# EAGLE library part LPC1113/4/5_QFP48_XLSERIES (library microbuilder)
LPC1113/4/5 ARM Cortex M0 MCU (50MHz) - XL Series (FBD48/3x3) LPC1115FBD48/303: Max Frequency: 50MHz Flash: 64kB SRAM: 8kB ADC: 10-bit
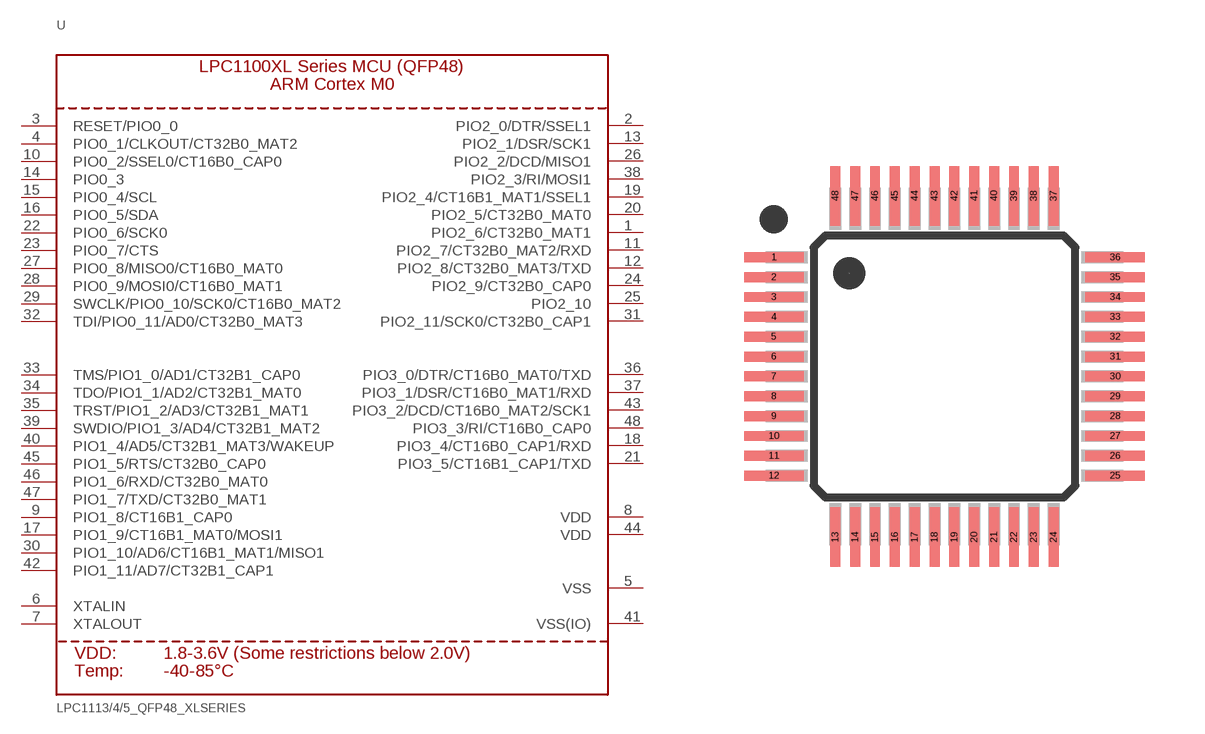
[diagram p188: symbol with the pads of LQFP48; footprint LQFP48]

Designator prefix U

## LPC1113/4/5_QFP48_XLSERIES  [LQFP48]
1  PIO2_6/CT32B0_MAT1
2  PIO2_0/DTR/SSEL1
3  RESET/PIO0_0
4  PIO0_1/CLKOUT/CT32B0_MAT2
5  VSS  pwr
6  XTALIN  in
7  XTALOUT  out
8  VDD  pwr
9  PIO1_8/CT16B1_CAP0
10  PIO0_2/SSEL0/CT16B0_CAP0
11  PIO2_7/CT32B0_MAT2/RXD
12  PIO2_8/CT32B0_MAT3/TXD
13  PIO2_1/DSR/SCK1
14  PIO0_3
15  PIO0_4/SCL
16  PIO0_5/SDA
17  PIO1_9/CT16B1_MAT0/MOSI1
18  PIO3_4/CT16B0_CAP1/RXD
19  PIO2_4/CT16B1_MAT1/SSEL1
20  PIO2_5/CT32B0_MAT0
21  PIO3_5/CT16B1_CAP1/TXD
22  PIO0_6/SCK0
23  PIO0_7/CTS
24  PIO2_9/CT32B0_CAP0
25  PIO2_10
26  PIO2_2/DCD/MISO1
27  PIO0_8/MISO0/CT16B0_MAT0
28  PIO0_9/MOSI0/CT16B0_MAT1
29  SWCLK/PIO0_10/SCK0/CT16B0_MAT2
30  PIO1_10/AD6/CT16B1_MAT1/MISO1
31  PIO2_11/SCK0/CT32B0_CAP1
32  TDI/PIO0_11/AD0/CT32B0_MAT3
33  TMS/PIO1_0/AD1/CT32B1_CAP0
34  TDO/PIO1_1/AD2/CT32B1_MAT0
35  TRST/PIO1_2/AD3/CT32B1_MAT1
36  PIO3_0/DTR/CT16B0_MAT0/TXD
37  PIO3_1/DSR/CT16B0_MAT1/RXD
38  PIO2_3/RI/MOSI1
39  SWDIO/PIO1_3/AD4/CT32B1_MAT2
40  PIO1_4/AD5/CT32B1_MAT3/WAKEUP
41  VSS(IO)  pwr
42  PIO1_11/AD7/CT32B1_CAP1
43  PIO3_2/DCD/CT16B0_MAT2/SCK1
44  VDD  pwr
45  PIO1_5/RTS/CT32B0_CAP0
46  PIO1_6/RXD/CT32B0_MAT0
47  PIO1_7/TXD/CT32B0_MAT1
48  PIO3_3/RI/CT16B0_CAP0

## Footprint LQFP48 (pad centres in mm)
smd 1.5 x 0.25: 1 -4.3,2.75; 2 -4.3,2.25; 3 -4.3,1.75; 4 -4.3,1.25; 5 -4.3,0.75; 6 -4.3,0.25; 7 -4.3,-0.25; 8 -4.3,-0.75; 9 -4.3,-1.25; 10 -4.3,-1.75; 11 -4.3,-2.25; 12 -4.3,-2.75; 25 4.3,-2.75; 26 4.3,-2.25; 27 4.3,-1.75; 28 4.3,-1.25; 29 4.3,-0.75; 30 4.3,-0.25; 31 4.3,0.25; 32 4.3,0.75; 33 4.3,1.25; 34 4.3,1.75; 35 4.3,2.25; 36 4.3,2.75
smd 0.25 x 1.5: 13 -2.75,-4.3; 14 -2.25,-4.3; 15 -1.75,-4.3; 16 -1.25,-4.3; 17 -0.75,-4.3; 18 -0.25,-4.3; 19 0.25,-4.3; 20 0.75,-4.3; 21 1.25,-4.3; 22 1.75,-4.3; 23 2.25,-4.3; 24 2.75,-4.3; 37 2.75,4.3; 38 2.25,4.3; 39 1.75,4.3; 40 1.25,4.3; 41 0.75,4.3; 42 0.25,4.3; 43 -0.25,4.3; 44 -0.75,4.3; 45 -1.25,4.3; 46 -1.75,4.3; 47 -2.25,4.3; 48 -2.75,4.3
